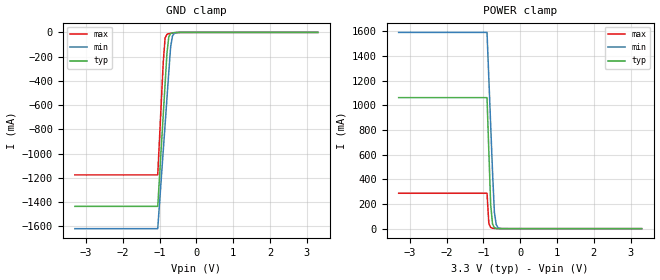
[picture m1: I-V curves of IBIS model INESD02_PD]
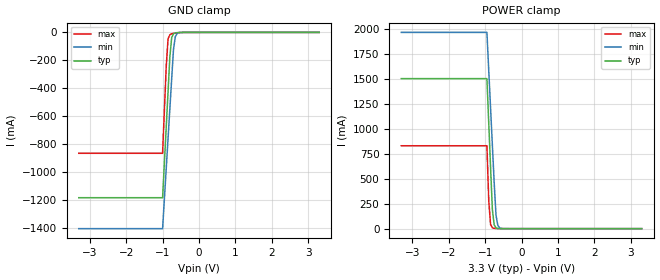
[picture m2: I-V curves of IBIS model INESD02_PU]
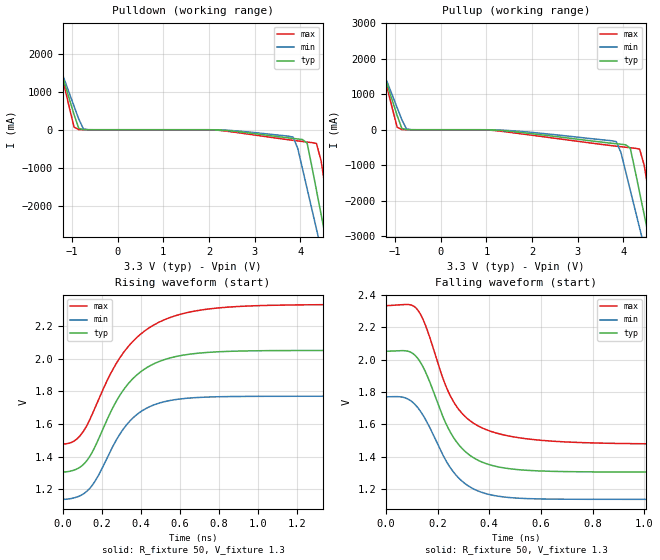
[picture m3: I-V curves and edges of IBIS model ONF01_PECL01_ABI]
|   This file is an IBIS representation of the   |
|   Integrated Device Technology, Inc.   |
|   ICS843202I   |
|  FEMTOCLOCKS 680MHZ, CRYSTAL-TO-3.3V DIF  LVPECL FREQUENCY SYNTHESIZER   |
[IBIS Ver]   4.1
[File name]   843202i_3v3.ibs
[File Rev]   1.1
[Date]   12 Jan 2009 | Last modified
|   Dec 30 2002 | Generated
[Source]   Originated at Integrated Devices Technology, Inc.
[Disclaimer]
IDT hereby grants the user of this IBIS model a non-exclusive,
nontransferable license to use this IBIS model under the following terms.
Before using this IBIS model, the user should read this license.
If the user does not accept these terms,  the IBIS model should be
returned to IDT within 30 days.
   The user is granted this license only to use the IBIS model and
is not granted rights to sell, load, rent, lease or license the IBIS
model in whole or in part, or in modified form to anyone other than
user. User may modify the IBIS model to suit its specific
applications but rights to derivative works and such modifications
shall belong to IDT.
   This IBIS model is provided on an "AS IS" basis and IDT makes
absolutely no warranty with respect to the information contained
herein. IDT DISCLAIMS AND CUSTOMER WAIVES ALL WARRANTIES, EXPRESS
OR IMPLIED, INCLUDING WARRANTIES OF MERCHANTABILITY OR FITNESS FOR
A PARTICULAR PURPOSE. The entire risk as to quality and performance
is with the Customer. ACCORDINGLY, IN NO EVENT SHALL THE COMPANY BE
LIABLE FOR ANY DAMAGES, WHETHER IN CONTRACT OR TORT,INCLUDING ANY
LOST PROFITS OR OTHER INCIDENTAL, CONSEQUENTIAL, EXEMPLARY, OR
PUNITIVE DAMAGES ARISING OUT OF THE USE OR APPLICATION OF THE IBIS
model provided in this package. Further, IDT reserves the right to
make changes without notice to any product herein to improve
reliability, function, or design. IDT does not convey any license
under patent rights or any other intellectual property rights,
including those of third parties.
   IDT is not obligated to provide maintenance or support
for the licensed IBIS model.
[Copyright]   Copyright 2008 by Integrated Device Technology, Inc.
[Component]   ICS843202YI
[Manufacturer] Integrated Devices Technology, Inc.
[Package]
|LQFP32
|lead + wire   typ   min   max
R_pkg   220.4m   212.5m   238m
L_pkg   1.841n   1.708n   1.974n
C_pkg   0.316p   0.2907p   0.33p
[Pin] signal_name  model_name   R_pin   L_pin   C_pin
1   VCCO_A   POWER   238m   1.974n   0.330p
2   NC   NC   225m   1.841n   0.311p
3   XTAL_IN1   NC   218m   1.7745n   0.301p
4   XTAL_OUT1  NC   213m   1.708n   0.291p
5   NC   NC   213m   1.708n   0.291p
6   REC_CLK   INESD02_PD   218m   1.7745n   0.301p
7   nREC_CLK   INESD02_PU   225m   1.841n   0.311p
8   VCCO_B   POWER   238m   1.974n   0.330p
9   NC   NC   238m   1.974n   0.330p
10   QB   ONF01_PECL01_ABI   225m   1.841n   0.311p
11   nQB   ONF01_PECL01_ABI   218m   1.7745n   0.301p
12   NC   NC   213m   1.708n   0.291p
13   NC   NC   213m   1.708n   0.291p
14   NC   NC   218m   1.7745n   0.301p
15   NC   NC   225m   1.841n   0.311p
16   VCCA   POWER   238m   1.974n   0.330p
17   SEL1   INESD02_PU_PECL   238m   1.974n   0.330p
18   VCC   POWER   225m   1.841n   0.311p
19   OEB   INESD02_PU   218m   1.7745n   0.301p
20   VEE   GND   213m   1.708n   0.291p
21   SEL0   INESD02_PD_PECL   213m   1.708n   0.291p
22   VCCA   POWER   218m   1.7745n   0.301p
23   VCC   POWER   225m   1.841n   0.311p
24   OEA   INESD02_PU   238m   1.974n   0.330p
25   VEE   GND   238m   1.974n   0.330p
26   NC   NC   225m   1.841n   0.311p
27   XTAL_OUT0  NC   218m   1.7745n   0.301p
28   XTAL_IN0   NC   213m   1.708n   0.291p
29   NC   NC   213m   1.708n   0.291p
30   nQA   ONF01_PECL01_ABI   218m   1.7745n   0.301p
31   QA   ONF01_PECL01_ABI   225m   1.841n   0.311p
32   NC   NC   238m   1.974n   0.330p
[Diff Pin]  inv_pin  vdiff tdelay_typ tdelay_min  tdelay_max
|Input
6   7  0.15 0  0  0
|Output
10   11   NA   0  0  0
31   30   NA   0  0  0
| Models and submodels in the file (5): INESD02_PD (Input), INESD02_PU (Input), ONF01_PECL01_ABI (Output_ECL), INESD02_PU_PECL (Input), INESD02_PD_PECL (Input)
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[Model]   INESD02_PD
Model_type   Input
Polarity   Non-Inverting
Vinl = 0.80V
Vinh = 2.0V
|   typ   min   max
C_comp   2pF   1.5pF   2.5pF
|   typ   min   max
[Voltage range]  3.3V   3.15V   3.45V
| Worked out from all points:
|   GND clamp passes 1 mA (typ) near -0.56 V on its own axis
|   POWER clamp passes 1 mA (typ) near -0.61 V on its own axis
[GND_clamp]
|Voltage   I(typ)   I(min)   I(max)
-3.3V     -1.436A    -1.62A     -1.176A
-1.05V    -1.436A    -1.62A     -1.176A
-900mV    -678.5mA   -975.1mA   -244mA
-850mV    -426.1mA   -760.1mA   -46.85mA
-800mV    -173.9mA   -545.4mA   -16.11mA
-750mV    -36.96mA   -330.7mA   -9.916mA
-700mV    -9.696mA   -120.2mA   -7.056mA
-650mV    -3.545mA   -29.7mA    -4.857mA
-600mV    -1.629mA   -7.52mA    -3.049mA
-400mV    -52.81uA   -52.52uA   -108.7uA
3.3V      71.13uA    77.43uA    62.11uA
[POWER_clamp]
|Voltage   I(typ)   I(min)   I(max)
-3.3V     1.063A     1.593A     287.3mA
-900mV    1.063A     1.593A     287.3mA
-850mV    620.5mA    1.215A     41.84mA
-800mV    191.6mA    837.5mA    8.757mA
-750mV    37.76mA    460.2mA    3.328mA
-700mV    8.104mA    133.8mA    1.728mA
-650mV    2.076mA    32.66mA    905.3uA
-600mV    678.1uA    8.083mA    443.8uA
-450mV    104.2uA    213.3uA    89.09uA
3.3V      -3.041nA   -3.986uA   0A
[Model]   INESD02_PU
Model_type   Input
Polarity   Non-Inverting
Vinl = 0.80V
Vinh = 2.0V
|   typ   min   max
C_comp   2pF   1.5pF   2.5pF
|   typ   min   max
[Voltage range]  3.3V   3.15V   3.45V
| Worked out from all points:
|   GND clamp passes 1 mA (typ) near -0.56 V on its own axis
|   POWER clamp passes 1 mA (typ) near -0.61 V on its own axis
[GND_clamp]
|Voltage   I(typ)   I(min)   I(max)
-3.3V     -1.184A    -1.405A    -865.6mA
-1V       -1.184A    -1.405A    -865.6mA
-900mV    -678.5mA   -975.1mA   -244.1mA
-850mV    -426.2mA   -760.2mA   -46.92mA
-800mV    -174mA     -545.4mA   -16.17mA
-750mV    -37.03mA   -330.8mA   -9.981mA
-700mV    -9.767mA   -120.3mA   -7.122mA
-650mV    -3.616mA   -29.78mA   -4.922mA
-600mV    -1.7mA     -7.594mA   -3.115mA
-400mV    -123.9uA   -126uA     -173.9uA
3.3V      1.866nA    3.949uA    0A
[POWER_clamp]
|Voltage   I(typ)   I(min)   I(max)
-3.3V     1.506A     1.97A      832.1mA
-950mV    1.506A     1.97A      832.1mA
-900mV    1.063A     1.592A     287.2mA
-850mV    620.4mA    1.215A     41.77mA
-800mV    191.5mA    837.4mA    8.692mA
-750mV    37.69mA    460.1mA    3.262mA
-700mV    8.032mA    133.8mA    1.662mA
-650mV    2.005mA    32.58mA    840.1uA
-600mV    607uA      8.009mA    378.6uA
-450mV    33.11uA    139.8uA    23.88uA
3.3V      -71.13uA   -77.46uA   -62.11uA
[Model]   ONF01_PECL01_ABI
Model_type  Output_ECL
Polarity   Non-Inverting
Vmeas = 1.63
Rref = 50
Cref = 0
Vref = 1.3
|Variable  typ   min   max
C_comp   2p   1.5p   2.5p
[Voltage Range]   3.3   3.135   3.465
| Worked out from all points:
|   rising waveform, R_fixture 50, V_fixture 1.3: 20-80 % time 218ps typ, 193ps min, 263ps max; typ from 1.31 V to 2.05 V
|   falling waveform, R_fixture 50, V_fixture 1.3: 20-80 % time 134ps typ, 136ps min, 142ps max; typ from 2.05 V to 1.31 V
| Open source, no load
|  Voltage   I(typ)   I(min)   I(max)
[Pulldown]
-3.3V     9.786A     8.425A     12.06A
-1.667V   3.247A     2.986A     3.704A
-1.463V   2.432A     2.308A     2.661A
-952.6mV  398mA      618.5mA    68.87mA
-850.5mV  36.63mA    281.6mA    4.032mA
3.844V    -229.1mA   -195.7mA   -279.4mA
4.151V    -352.7mA   -1.559A    -324.9mA
4.355V    -1.599A    -2.62A     -360.9mA
4.559V    -2.871A    -3.681A    -1.635A
4.661V    -3.508A    -4.211A    -2.446A
4.763V    -4.144A    -4.742A    -3.257A
6.6V      -15.69A    -14.35A    -17.99A
[Pullup]
-3.3V     9.786A     8.425A     12.06A
-1.565V   2.839A     2.647A     3.182A
-952.6mV  398mA      618.5mA    68.87mA
-850.5mV  36.63mA    281.6mA    4.032mA
-646.4mV  229.3uA    964.8uA    177.5uA
3.844V    -394.4mA   -337mA     -463.1mA
4.151V    -517.8mA   -1.701A    -507.4mA
4.355V    -1.764A    -2.763A    -542.7mA
4.559V    -3.036A    -3.825A    -1.816A
4.661V    -3.672A    -4.355A    -2.626A
4.763V    -4.308A    -4.886A    -3.437A
6.6V      -15.79A    -14.46A    -18.06A
[Ramp]
|   typ   min   max
dV/dt_r   0.596/0.354n   0.506/0.311n   0.684/0.427n
dV/dt_f   0.599/0.219n   0.507/0.219n   0.690/0.252n
R_load =   50.0000
[Rising Waveform]
R_fixture = 50
V_fixture = 1.3   | VCC_typ - 2V
V_fixture_max = 1.465   | VCC_max - 2V
V_fixture_min = 1.135   | VCC_min - 2V
C_fixture = 0.0p
| Time   typ   min   max
0s        1.306V     1.138V     1.478V
67.2ps    1.321V     1.15V      1.503V
126ps     1.379V     1.19V      1.597V
176.4ps   1.489V     1.271V     1.731V
247.8ps   1.679V     1.442V     1.915V
338.1ps   1.85V      1.61V      2.079V
430.5ps   1.946V     1.698V     2.18V
554.4ps   2.007V     1.745V     2.255V
936.6ps   2.049V     1.77V      2.324V
1.999ns   2.052V     1.771V     2.333V
[Falling Waveform]
R_fixture = 50
V_fixture = 1.3   | VCC_typ - 2V
V_fixture_max = 1.465   | VCC_max - 2V
V_fixture_min = 1.135   | VCC_min - 2V
C_fixture = 0.0p
| Time   typ   min   max
0s        2.052V     1.771V     2.334V
73.5ps    2.055V     1.765V     2.34V
119.7ps   2.015V     1.711V     2.314V
151.2ps   1.932V     1.637V     2.221V
224.7ps   1.633V     1.399V     1.868V
268.8ps   1.503V     1.293V     1.723V
336ps     1.398V     1.205V     1.611V
434.7ps   1.338V     1.157V     1.544V
806.4ps   1.307V     1.138V     1.486V
1.999ns   1.306V     1.138V     1.478V
